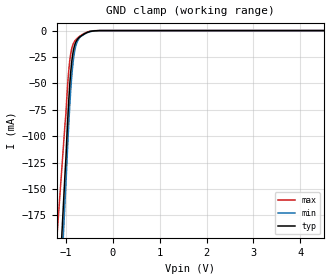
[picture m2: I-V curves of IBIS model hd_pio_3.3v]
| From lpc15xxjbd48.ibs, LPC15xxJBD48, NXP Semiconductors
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[Model] hd_pio_3.3v
Model_type Input
Vinl = 990.000mV
Vinh = 2.31000V
C_comp 1.52000pF 1.52000pF 1.52000pF
| variable typ   min   max
[Voltage Range] 3.30000V 3.00000V 3.60000V
[POWER Clamp Reference] 3.30000V 3.00000V 3.60000V
[GND Clamp Reference] 0.00000V 0.00000V 0.00000V
[Temperature Range]   25   85   -40
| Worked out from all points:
|   GND clamp passes 1 mA (typ) near -0.49 V on its own axis
[GND Clamp]
-3.3V     -2.092A    -2.24A     -1.503A
-1.02V    -136.5mA   -162.9mA   -89.08mA
-1V       -121mA     -145.6mA   -78.71mA
-960mV    -83.35mA   -107.1mA   -49.72mA
-920mV    -52.59mA   -72.89mA   -29.28mA
-880mV    -31.29mA   -46.03mA   -17.86mA
-840mV    -18.71mA   -27.63mA   -12.25mA
-800mV    -12.16mA   -16.61mA   -9.308mA
-740mV    -7.606mA   -8.868mA   -6.601mA
-560mV    -2.076mA   -2.347mA   -1.597mA
-280mV    0A         0A         0A
6.6V      0A         0A         0A
[POWER Clamp]
-3.3V     0A         0A         0A
6.6V      0A         0A         0A
